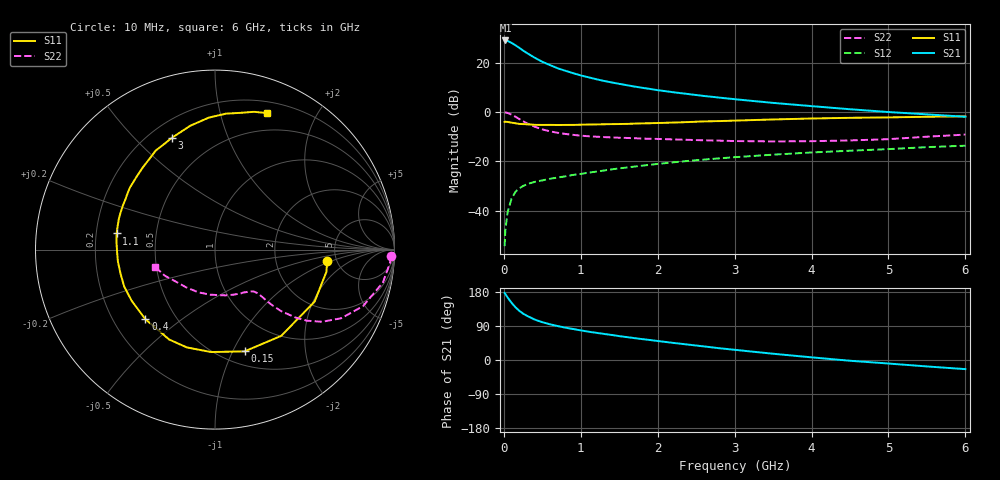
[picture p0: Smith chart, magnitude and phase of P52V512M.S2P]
! SIEMENS Small Signal Semiconductors
! BFP183
! Si NPN RF Bipolar Junction Transistor in SOT143
! VCE = 2.5 V  IC = 12 mA
! Common Emitter S-Parameters:  March  1996
# GHz  S  MA  R  50
!  f  S11  S21  S12  S22
! GHz  MAG  ANG  MAG  ANG  MAG  ANG  MAG  ANG
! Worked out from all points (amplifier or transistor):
!   36 points, 10 MHz to 6 GHz, reference 50 ohm
!   highest |S21| = 29.0 dB at 20 MHz (marker M1)
!   |S21| within 3 dB of that: start of sweep to 201.8 MHz
!   unconditionally stable (mu >= 1): 1.033 GHz to 5.495 GHz
!   at 250 MHz: K = 0.37, MSG = 27.5 dB, |S12| = -30.0 dB
!   at 1.4 GHz: K = 1.10, MAG = 15.7 dB, |S12| = -23.3 dB
!   at 6 GHz: K = 0.97, MSG = 5.9 dB, |S12| = -13.7 dB
!   S11 on the Smith chart (normalised r, x): 10 MHz: 4.20, -0.85; 150 MHz: 0.64, -1.11; 400 MHz: 0.34, -0.37; 1.1 GHz: 0.29, +0.07; 3 GHz: 0.29, +0.64; 6 GHz: 0.31, +1.40
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0.01  0.6283 -5.6  28.12 177.0  0.0019 79.8  0.9798 -2.2
0.02  0.633 -11.3  28.12 174.1  0.0041 80.2  0.9773 -4.5
0.05  0.626 -27.6  27.48 164.7  0.0095 80.8  0.9533 -11.1
0.1  0.6059 -52.5  25.12 151.0  0.0174 67.4  0.8828 -20.9
0.15  0.5905 -73.8  22.49 139.3  0.0239 60.0  0.801 -28.5
0.2  0.5712 -92.2  20 129.9  0.0282 54.8  0.7192 -34.0
0.25  0.5671 -106.1  17.57 122.4  0.0315 50.4  0.6479 -37.7
0.3  0.5623 -117.0  15.64 116.7  0.0343 48.3  0.5886 -40.1
0.4  0.5485 -135.0  12.6 106.8  0.0382 44.6  0.5023 -43.0
0.5  0.5448 -148.3  10.39 99.8  0.0409 42.9  0.4433 -44.2
0.6  0.5462 -157.9  8.909 94.2  0.0442 43.6  0.4043 -44.8
0.7  0.5432 -166.0  7.681 89.5  0.0468 43.9  0.3774 -45.0
0.9  0.5458 -178.8  6.112 81.8  0.0529 44.7  0.3429 -45.6
1.1  0.5556 170.7  5.034 74.7  0.0587 45.8  0.3215 -46.9
1.5  0.5688 154.6  3.708 63.0  0.0717 46.1  0.3002 -51.1
1.8  0.5866 143.9  3.088 55.1  0.0815 46.2  0.2884 -55.7
2.2  0.6086 131.7  2.511 45.2  0.095 44.5  0.2772 -63.0
3  0.667 111.3  1.812 26.9  0.1209 39.5  0.2569 -82.0
3.5  0.7036 101.3  1.525 16.5  0.1362 36.0  0.2525 -95.8
4.5  0.7598 85.4  1.134 -2.0  0.1636 28.0  0.2644 -127.0
5.5  0.7978 74.2  0.893 -17.0  0.1935 20.8  0.3147 -152.4
6  0.814 69.2  0.798 -24.1  0.2068 16.5  0.3473 -163.7
